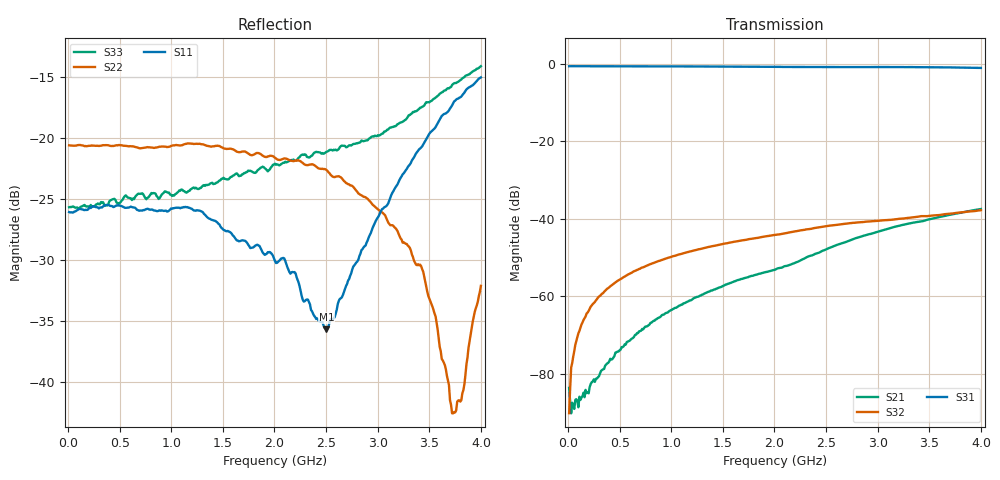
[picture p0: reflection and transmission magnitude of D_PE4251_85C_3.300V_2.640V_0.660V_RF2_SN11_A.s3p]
! Device ID: PE4251_SoldCshunt_081809
! Dir: c:\Test Bench Repositories\Bench_Software_CVI_Version_8\trunk\PSC 4Port_VNA Bench\datalog\4250\TEST\PE4251_SoldCshunt_081809\85C\3p300000\RF2
! Serial: 11
! Insertion: A
! Temp: 85C
! VDD: 3.300
! Control_Hi: 80.000
! Control_Lo: 20.000
! Logic State: RF2
! Port 1: RFC
! Port 2: RF1
! Port 3: RF2
! V1 = 0.66
! V2 = 0.66
! V3 = 0.66
! IDD: 4.660040e-05
! FILE NAME
! DATE 08/18/09  20:17
! CORRECTED  DATA
#  Hz  S  RI  R  50.00
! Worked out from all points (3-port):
!   401 points, 10 MHz to 4 GHz, reference 50 ohm
!   strongest paths, dB at 10 MHz, 1.008 GHz, 2.005 GHz, 3.002 GHz, 4 GHz:
!     S31: -0.6, -0.7, -0.8, -0.8, -1.1
!     S32: -90.1, -49.7, -44.1, -40.5, -37.8
!     S21: -83.6, -63.4, -53.1, -43.3, -37.5
!   lowest |S11| = -35.6 dB at 2.504 GHz (marker M1), VSWR 1.03, Z = 50.4 - j1.61 ohm
!   |S11| at or under -10 dB: start of sweep to end of sweep
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1e7  0.0499 -0.000764  8.45e-05 -4.06e-05  0.9308 -0.00354
     -3.05e-06 -6.59e-05  0.0937 -0.000958  7.23e-05 -7.15e-06
     0.9314 -0.00494  1.32e-05 2.82e-05  0.0522 0.000655
1.696e8  0.051 0.000191  -2.9e-06 -4.65e-05  0.9292 -0.0593
         6.67e-06 -6.18e-05  0.093 -0.00374  5.39e-05 0.000557
         0.93 -0.0598  5.94e-05 0.000547  0.0528 6.22e-05
3.19225e8  0.0521 -0.00165  -4.97e-05 -8.87e-05  0.9229 -0.1117
           -4.31e-05 -0.000101  0.093 -0.00826  8.93e-05 0.00105
           0.9244 -0.1106  8.78e-05 0.00105  0.0548 -0.00312
4.98775e8  0.0529 -0.00364  -0.000151 -0.000124  0.9128 -0.1714
           -0.000153 -0.000131  0.0932 -0.012  0.000155 0.00163
           0.9129 -0.1714  0.000158 0.00164  0.0541 -0.00471
1.037425e9  0.0501 -0.0137  -0.000689 -0.000156  0.8597 -0.3456
            -0.000695 -0.000148  0.0901 -0.0266  0.000474 0.00332
            0.86 -0.3452  0.000465 0.00331  0.0576 -0.0131
2.005e9  0.0306 -0.00721  -0.00221 -7.1e-05  0.6875 -0.603
         -0.00221 -7.34e-05  0.0768 -0.0324  0.00103 0.00612
         0.6879 -0.6021  0.00105 0.00614  0.069 -0.0381
2.50375e9  0.00447 -0.0159  -0.00404 -0.00039  0.5769 -0.6997
           -0.00404 -0.000399  0.0681 -0.0296  0.00139 0.00792
           0.5786 -0.6995  0.00137 0.00794  0.0509 -0.0721
3.42145e9  -0.0828 -0.0398  -0.00907 0.00195  0.3249 -0.845
           -0.00906 0.00191  0.0242 -0.0177  0.00202 0.0106
           0.3292 -0.8444  0.00202 0.0107  -0.0361 -0.129
3.74065e9  -0.1362 -0.0395  -0.011 0.00349  0.2161 -0.871
           -0.011 0.00346  -0.00099 -0.0075  0.00188 0.0117
           0.2166 -0.8705  0.00189 0.0117  -0.0921 -0.1409
4e9  -0.1752 -0.0312  -0.0125 0.00504  0.1203 -0.8788
     -0.0124 0.00501  -0.0248 -0.00226  0.00196 0.0127
     0.122 -0.8776  0.00195 0.0128  -0.1415 -0.1383
